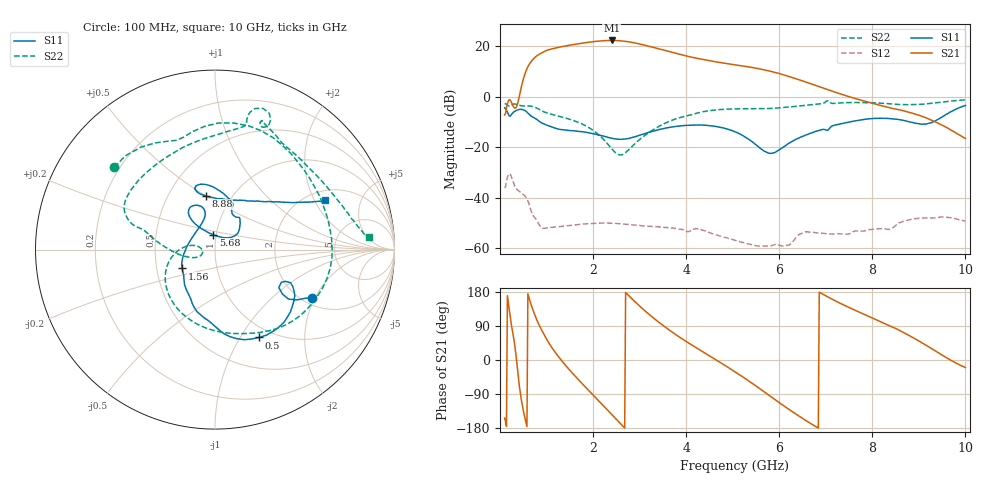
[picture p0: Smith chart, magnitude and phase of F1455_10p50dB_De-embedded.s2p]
! Integrated Device Technology
! Corporate Headquarters
! 6024 Silver Creek Valley Road
! San Jose, CA 95138  USA
! Phone:  1-408-284-8200
! Toll Free:  1-800-223-1366
! Webpage:  http://www.idt.com/
! Timing and RF Division
! 515 Groton Road, Suite 102
! Westford, MA 01886-6024
! Device:  F1455
! Description: 6-bit 0.5 dB Transmit Variable Gain Amplifier
! Frequency:  1400.0 -  2300.00 MHz
! Package:  6x6 mm Thin QFN Plastic Package: 28 pin
! State:  21
! Atten State:  10.5 dB
! Voltage:  +5.00 Volts
! Current:  217.652 mA
! Data:  The device was measured on a the F1455 evaluation board which has
!  individual transmission lines to the RF pins.  Data was collected
!  using a calibrated network analyzer.  The evaluation board was
!  de-embedded using a TRL calibration technique.
!  The reference plane is the edge of the package pin.
!  Pin  1 = CSb
!  Pin  2 = DATA
!  Pin  3 = CLK
!  Pin  4 = RSET
!  Pin  5 = GND
!  Pin  6 = RFIN  = Port 1
!  Pin  7 = GND
!  Pin  8 = NC
!  Pin  9 = NC
!  Pin 10 = NC
!  Pin 11 = NC
!  Pin 12 = NC
!  Pin 13 = NC
!  Pin 14 = /STBY
!  Pin 15 = GND
!  Pin 16 = RFOUT  = Port 2
!  Pin 17 = GND
!  Pin 18 = NC
!  Pin 19 = NC
!  Pin 20 = NC
!  Pin 21 = GND
!  Pin 22 = NC
!  Pin 23 = GND
!  Pin 24 = NC
!  Pin 25 = NC
!  Pin 26 = NC
!  Pin 27 = GND
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# GHz S dB R 50
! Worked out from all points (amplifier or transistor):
!   496 points, 100 MHz to 10 GHz, reference 50 ohm
!   highest |S21| = 22.3 dB at 2.4 GHz (marker M1)
!   |S21| within 3 dB of that: 1.193 GHz to 3.351 GHz (2.158 GHz wide, 95 % of centre)
!   unconditionally stable (mu >= 1): start of sweep to end of sweep
!   at 1.74 GHz: K = 12.94, MAG = 21.7 dB, |S12| = -50.5 dB
!   at 5.06 GHz: K = 53.66, MAG = 14.5 dB, |S12| = -57.0 dB
!   at 10 GHz: K = 137.98, MAG = -8.1 dB, |S12| = -49.2 dB
!   S11 on the Smith chart (normalised r, x): 100 MHz: 2.23, -1.88; 500 MHz: 0.87, -1.21; 1.56 GHz: 0.68, -0.15; 5.68 GHz: 0.97, +0.16; 8.88 GHz: 0.76, +0.50; 10 GHz: 2.44, +2.43
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0.1  -4.42 -26.5  -7.22 -153.3  -36.21 44.5  -2.80 140.8
0.38  -5.26 -39.8  -2.80 -28.6  -37.02 -112.2  -3.22 56.8
0.5  -5.23 -63.3  6.79 -132.2  -38.76 -150.7  -3.68 28.0
0.68  -7.81 -93.4  14.11 142.2  -45.81 147.0  -3.81 -14.1
0.8  -9.15 -108.5  16.29 103.4  -49.28 131.2  -4.60 -42.2
0.94  -10.79 -120.7  17.77 68.9  -52.17 124.3  -5.98 -68.4
1.24  -12.78 -139.3  19.45 11.6  -51.57 92.0  -7.66 -110.0
1.56  -13.53 -150.0  20.59 -35.2  -50.96 61.7  -9.34 -142.8
1.76  -13.88 -156.6  21.17 -61.6  -50.52 46.4  -10.79 -159.3
2.08  -14.98 -170.5  21.94 -102.4  -50.18 24.8  -14.48 178.3
2.4  -16.49 165.4  22.26 -143.6  -50.15 5.2  -20.62 169.9
2.58  -16.89 147.2  22.12 -166.8  -50.36 -4.7  -23.13 -172.9
2.76  -16.61 129.6  21.74 170.7  -50.64 -13.0  -21.14 -157.4
3.06  -14.97 110.2  20.61 135.7  -51.18 -25.9  -16.12 -164.5
3.4  -13.14 104.9  19.02 101.0  -51.60 -38.4  -11.96 -179.9
4.08  -11.34 114.8  15.78 42.7  -53.35 -58.2  -7.32 164.1
5.06  -14.00 128.2  12.60 -31.9  -57.02 -98.9  -4.85 148.7
5.68  -21.64 96.5  10.61 -84.1  -59.25 -100.5  -4.77 123.3
6.7  -14.37 43.7  4.97 -169.4  -53.71 -139.2  -3.19 78.5
8.36  -8.67 106.9  -4.34 90.8  -52.56 160.2  -2.82 62.4
8.88  -10.34 100.0  -6.69 58.7  -48.48 143.1  -3.18 41.9
10  -3.48 24.1  -16.57 -19.9  -49.25 70.2  -1.29 4.6
